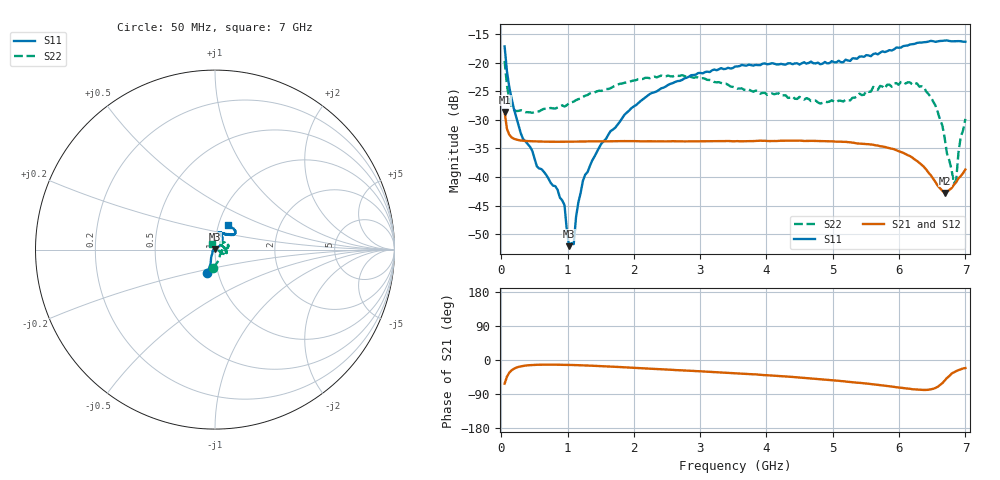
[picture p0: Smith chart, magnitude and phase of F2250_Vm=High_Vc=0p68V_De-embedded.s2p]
! Integrated Device Technology
! Corporate Headquarters
! 6024 Silver Creek Valley Road
! San Jose, CA 95138  USA
! Phone:  1-408-284-8200
! Toll Free:  1-800-223-1366
! Webpage:  http://www.idt.com/
! Timing and RF Division
! 515 Groton Road, Suite 102
! Westford, MA 01886-6024
! Device:  F2250
! Description: Voltage Variable RF Attenuator
! Frequency:  50.0 -  6000.00 MHz
! Package:  3x3 mm Thin QFN Plastic Package: 16 pin
! Ports:  2 RF, 3 DC
!  Pin  1  = GND
!  Pin  2  = NC
!  Pin  3  = RF1  = Port 1
!  Pin  4  = NC
!  Pin  5  = GND
!  Pin  6  = GND
!  Pin  7  = GND
!  Pin  8  = GND
!  Pin  9  = NC
!  Pin 10  = RF2  = Port 2
!  Pin 11  = NC
!  Pin 12  = GND
!  Pin 13  = GND
!  Pin 14  = VCNTRL
!  Pin 15  = VDD
!  Pin 16  = VMODE
! Vcntrl:  0.680 Volts
! Vmode:  +3.300 Volts
! Vdd:  +3.30  Volts
! Current:  1.284 mA
! Data:  The device was measured on a the F2250 evaluation board which has
!  individual transmission lines to the RF pins.  Data was collected
!  using a calibrated network analyzer.  The evaluation board was
!  de-embedded using a TRL calibration technique.
!  The reference plane is the edge of the package pin.
! Misc:  SN 10
!  Action Tracker AT0258
! Date Measured:  2014-11-26
! Date:  2015-10-15  MJV
! Note:
!  Integrated Device Technology supplies this data as a sample of measured
!  data at the package pin for this product.  Your particular data for this
!  product may vary.
!  Data was taken at 25 degrees C.
!  Integrated Device Technology reserves the right to change this data at anytime.
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# GHz S dB R 50
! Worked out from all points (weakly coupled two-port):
!   201 points, 50 MHz to 7 GHz, reference 50 ohm
!   highest |S21| = -28.61 dB at 50 MHz (marker M1); lowest = -42.8 dB at 6.687 GHz (marker M2)
!   lowest |S11| = -52.1 dB at 1.023 GHz (marker M3), VSWR 1.00, Z = 49.8 + j0.171 ohm
!   |S11| at or under -10 dB: start of sweep to end of sweep
!   |S22| runs from -41.2 to -19.7 dB; largest |S21 - S12| = 6.3e-05
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0.05  -17.16 -108.2  -28.61 -62.5  -28.61 -62.4  -19.69 -95.0
0.1195  -24.20 -111.5  -32.59 -33.7  -32.59 -33.7  -26.41 -57.7
0.189  -28.01 -119.3  -33.31 -23.2  -33.30 -23.2  -28.23 -39.8
0.5365  -38.14 -153.2  -33.78 -12.7  -33.78 -12.7  -28.54 -9.0
0.9535  -44.91 171.5  -33.84 -12.7  -33.84 -12.7  -27.68 -3.9
1.023  -52.10 136.3  -33.83 -13.0  -33.83 -13.0  -27.08 -2.7
1.0925  -51.74 79.4  -33.83 -13.3  -33.83 -13.3  -26.82 -1.7
1.12725  -47.02 55.1  -33.82 -13.5  -33.82 -13.5  -26.54 -2.2
1.2315  -40.64 37.9  -33.79 -14.1  -33.80 -14.1  -25.99 -2.7
1.6485  -31.97 40.2  -33.75 -17.4  -33.75 -17.4  -24.46 3.7
2.37825  -24.75 46.2  -33.76 -24.1  -33.76 -24.1  -22.42 13.4
3.525  -20.68 71.5  -33.75 -35.0  -33.75 -35.0  -24.33 39.4
4.7065  -20.09 71.9  -33.68 -49.1  -33.68 -49.1  -26.63 46.1
5.2625  -19.69 53.0  -33.93 -58.1  -33.93 -58.1  -26.60 19.5
5.85325  -17.81 40.4  -34.96 -69.3  -34.96 -69.4  -23.83 -7.0
6.3745  -16.42 40.8  -38.22 -79.1  -38.24 -79.1  -24.27 -23.5
6.54825  -16.36 44.6  -40.88 -73.8  -40.89 -73.9  -27.50 -28.8
6.68725  -16.13 47.7  -42.79 -54.4  -42.79 -54.3  -33.16 -15.0
6.82625  -16.25 52.4  -41.38 -32.6  -41.36 -32.6  -41.17 62.2
6.861  -16.24 54.4  -40.91 -29.3  -40.89 -29.2  -40.56 76.3
6.9305  -16.25 58.6  -39.84 -24.6  -39.82 -24.7  -32.96 111.3
7  -16.35 62.3  -38.69 -21.2  -38.67 -21.3  -29.83 117.4
